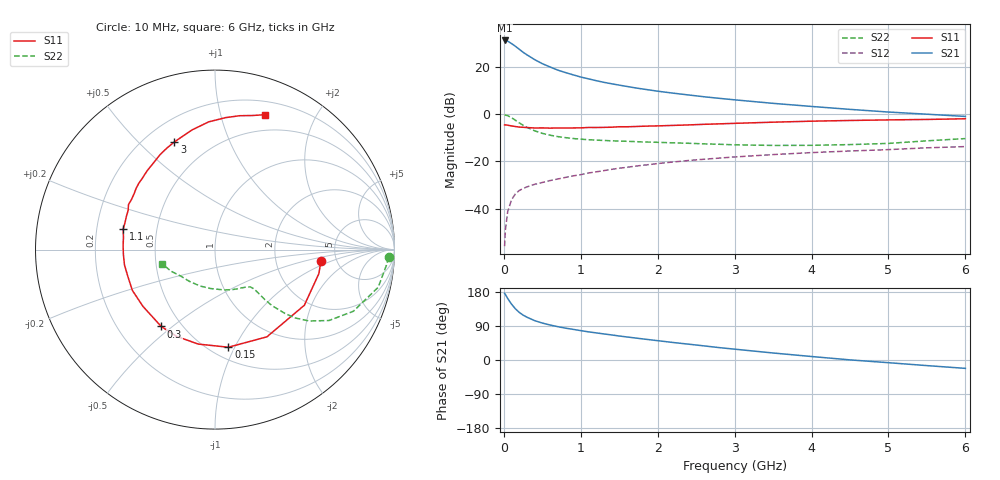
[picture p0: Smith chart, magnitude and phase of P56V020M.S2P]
! SIEMENS Small Signal Semiconductors
! BFP183
! Si NPN RF Bipolar Junction Transistor in SOT143
! VCE = 6 V  IC = 20 mA
! Common Emitter S-Parameters:  March  1996
# GHz  S  MA  R  50
!  f  S11  S21  S12  S22
! GHz  MAG  ANG  MAG  ANG  MAG  ANG  MAG  ANG
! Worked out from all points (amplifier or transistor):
!   36 points, 10 MHz to 6 GHz, reference 50 ohm
!   highest |S21| = 31.3 dB at 10 MHz (marker M1)
!   |S21| within 3 dB of that: start of sweep to 171.2 MHz
!   unconditionally stable (mu >= 1): 898.3 MHz to 5.704 GHz
!   at 250 MHz: K = 0.45, MSG = 28.9 dB, |S12| = -31.5 dB
!   at 1.4 GHz: K = 1.11, MAG = 16.1 dB, |S12| = -23.4 dB
!   at 6 GHz: K = 0.96, MSG = 6.4 dB, |S12| = -13.7 dB
!   S11 on the Smith chart (normalised r, x): 10 MHz: 3.76, -0.74; 150 MHz: 0.61, -0.94; 300 MHz: 0.39, -0.46; 1.1 GHz: 0.32, +0.10; 3 GHz: 0.32, +0.64; 6 GHz: 0.33, +1.39
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0.01  0.5935 -6.2  36.61 176.0  0.0016 85.4  0.969 -2.5
0.02  0.594 -13.0  36.59 172.9  0.0035 78.8  0.9592 -5.2
0.05  0.5865 -31.9  35.37 162.3  0.0086 79.2  0.9332 -13.0
0.1  0.5656 -59.2  31.47 147.4  0.0154 64.5  0.8443 -24.0
0.15  0.549 -82.2  27.55 135.1  0.0205 58.8  0.7479 -31.9
0.2  0.5346 -100.1  23.86 125.7  0.0242 55.2  0.6579 -37.2
0.25  0.5287 -113.9  20.6 118.5  0.0266 51.5  0.5861 -40.5
0.3  0.5226 -125.0  18.17 113.0  0.0289 49.3  0.5272 -42.4
0.4  0.511 -141.7  14.38 103.9  0.0327 48.3  0.4459 -44.5
0.5  0.5134 -153.7  11.79 97.5  0.0358 48.4  0.3937 -45.1
0.6  0.5081 -162.8  10.05 92.4  0.0393 49.0  0.3597 -45.1
0.7  0.5116 -170.4  8.626 88.0  0.0424 49.9  0.3358 -45.1
0.8  0.5111 -176.9  7.652 84.1  0.0458 50.7  0.3196 -45.2
1  0.5147 172.2  6.149 77.5  0.0524 51.7  0.2964 -45.9
1.1  0.5244 167.4  5.625 74.3  0.0568 51.8  0.2882 -46.4
1.5  0.5433 152.5  4.139 63.3  0.0718 51.5  0.27 -50.5
2.2  0.58 130.5  2.799 46.2  0.0973 47.6  0.2476 -62.8
3  0.6414 110.6  2.02 28.6  0.1243 41.0  0.2248 -82.1
3.5  0.6788 100.9  1.702 18.5  0.1397 36.8  0.2184 -96.7
4.5  0.7377 85.4  1.268 0.3  0.1663 27.8  0.2273 -128.9
5.5  0.7756 74.4  1.002 -14.8  0.1944 20.3  0.2734 -154.0
6  0.802 69.6  0.898 -22.1  0.2061 15.7  0.3048 -165.0
